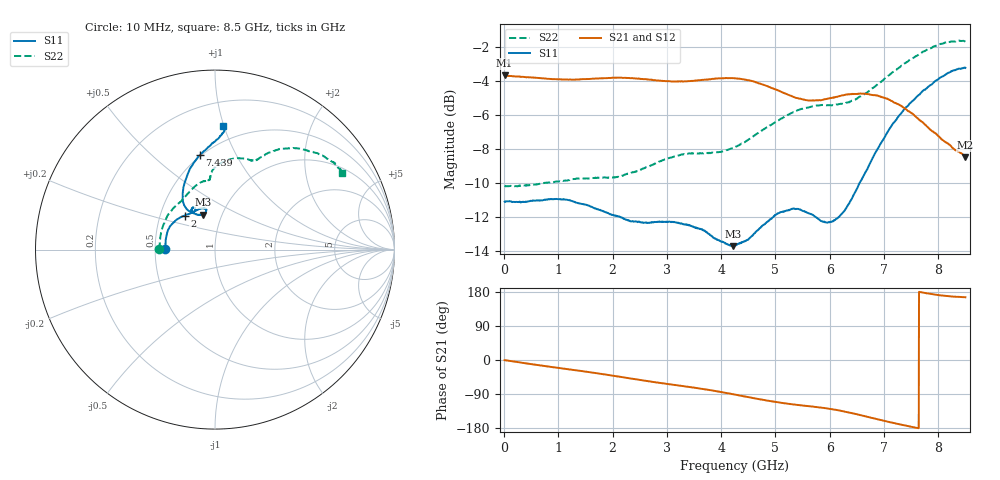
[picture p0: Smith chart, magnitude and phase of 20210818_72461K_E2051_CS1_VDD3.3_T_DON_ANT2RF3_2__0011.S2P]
!Agilent Technologies,E5071C,MY46417908,A.11.23
!Date: Wed Aug 18 14:30:50 2021
!Data & Calibration Information:
!Freq	S11:SOLT2(ON)	S21:SOLT2(ON)	S12:SOLT2(ON)	S22:SOLT2(ON)
!PortZ  Port1:50+j0  Port2:50+j0
!Above PortZ is port z conversion or system Z0 setting when saving the data.
!When reading, reference impedance value at option line is always used.
# Hz S dB R 50
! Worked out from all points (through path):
!   1601 points, 10 MHz to 8.5 GHz, reference 50 ohm
!   highest |S21| = -3.68 dB at 10 MHz (marker M1); lowest = -8.5 dB at 8.5 GHz (marker M2)
!   group delay of S21, straight-line fit = 65 ps
!   lowest |S11| = -13.7 dB at 4.213 GHz (marker M3), VSWR 1.52, Z = 40.7 + j16.5 ohm
!   |S11| at or under -10 dB: start of sweep to 6.552 GHz
!   |S22| runs from -10.2 to -1.6 dB; largest |S21 - S12| = 0.004
!   S11 on the Smith chart (normalised r, x): 10 MHz: 0.56, +0.00; 2 GHz: 0.67, +0.27; 7.439 GHz: 0.49, +0.73; 8.5 GHz: 0.38, +0.99
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1e7  -11.11 179.6  -3.68 -0.4  -3.68 -0.4  -10.17 179.8
8.536938e8  -10.95 160.4  -3.88 -18.0  -3.88 -18.0  -9.97 158.2
1.426769e9  -11.24 145.3  -3.90 -29.2  -3.90 -29.2  -9.74 141.7
1.999844e9  -11.90 131.8  -3.81 -41.2  -3.81 -41.2  -9.68 127.5
2.403119e9  -12.28 122.9  -3.85 -50.4  -3.85 -50.4  -9.37 118.5
2.843538e9  -12.30 113.9  -3.98 -59.9  -3.97 -59.9  -8.79 109.5
3.597025e9  -12.71 102.2  -3.96 -75.1  -3.96 -75.1  -8.28 97.4
4.21255e9  -13.74 108.9  -3.84 -90.2  -3.83 -90.2  -7.95 94.0
4.255e9  -13.69 109.7  -3.84 -91.3  -3.84 -91.3  -7.90 93.7
4.562762e9  -13.13 117.4  -4.00 -99.6  -4.00 -99.6  -7.33 92.6
4.918281e9  -12.12 121.0  -4.40 -108.7  -4.40 -108.6  -6.60 88.5
5.321556e9  -11.53 118.3  -4.93 -117.1  -4.93 -117.1  -5.85 80.6
5.671769e9  -11.87 115.9  -5.15 -122.7  -5.17 -122.8  -5.51 73.4
6.032594e9  -12.30 119.6  -5.00 -129.6  -5.01 -129.8  -5.44 68.3
6.3775e9  -11.09 125.0  -4.78 -139.1  -4.76 -139.3  -5.22 65.3
6.738325e9  -8.88 120.0  -4.80 -151.5  -4.78 -151.6  -4.56 62.4
7.088538e9  -6.89 109.3  -5.09 -163.5  -5.10 -163.5  -3.67 58.1
7.43875e9  -5.46 99.1  -5.76 -174.2  -5.76 -174.3  -2.86 51.6
7.714675e9  -4.59 91.8  -6.44 178.0  -6.44 177.9  -2.28 45.2
8.022438e9  -3.82 86.7  -7.30 170.8  -7.25 170.9  -1.84 38.4
8.351425e9  -3.31 85.7  -8.14 166.8  -8.10 166.9  -1.63 32.8
8.5e9  -3.23 86.3  -8.49 165.5  -8.41 165.7  -1.69 31.1
